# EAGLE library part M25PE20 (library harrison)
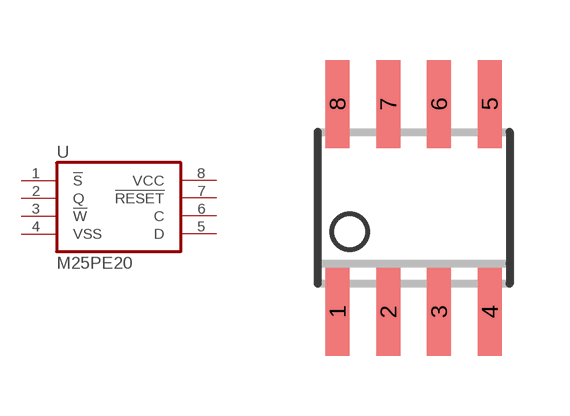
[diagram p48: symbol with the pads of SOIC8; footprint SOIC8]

Designator prefix U

## M25PE20  [SOIC8]
1  !S!  in
2  Q  out
3  !W!  in
4  VSS  pwr
5  D  in
6  C  in
7  !RESET!  in
8  VCC  pwr

## Footprint SOIC8 (pad centres in mm)
smd 0.6 x 2.2: 1 -1.905,-2.6; 2 -0.635,-2.6; 3 0.635,-2.6; 4 1.905,-2.6; 5 1.905,2.6; 6 0.635,2.6; 7 -0.635,2.6; 8 -1.905,2.6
